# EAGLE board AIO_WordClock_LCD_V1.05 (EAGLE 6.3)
PROJECT_AUTHOR: C. Wille; PROJECT_COPYRIGHT: (c) 11/2012; PROJECT_REVISION: V1.05
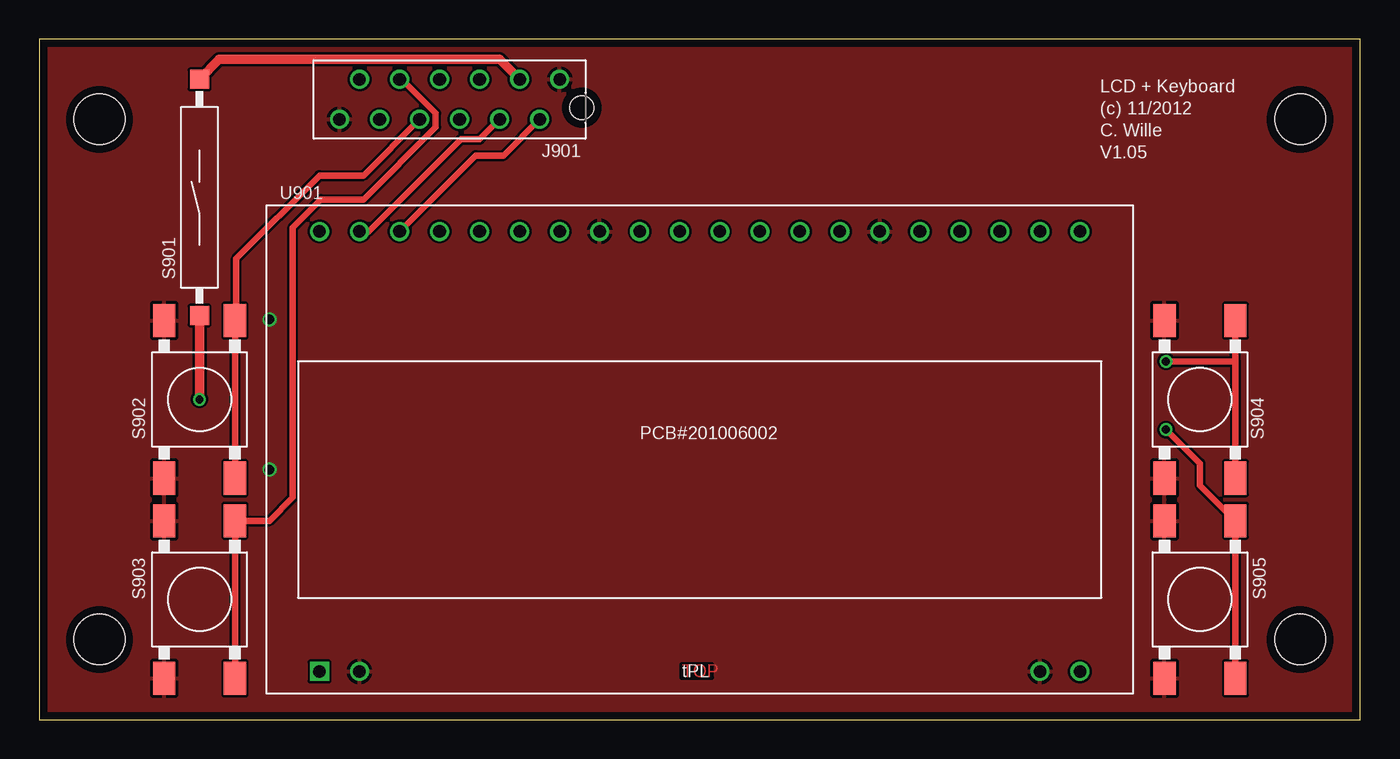
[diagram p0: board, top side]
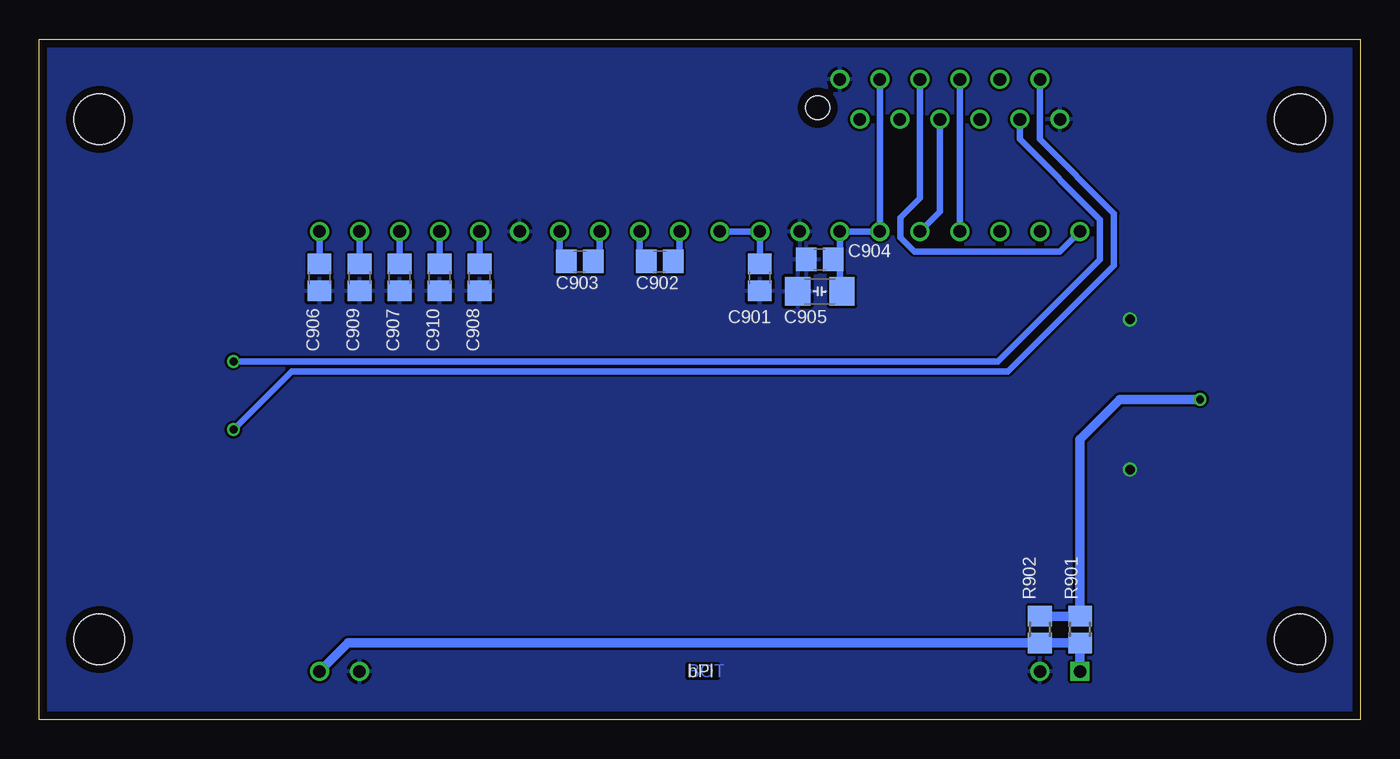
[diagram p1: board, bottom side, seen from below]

Size 83.82 x 43.18 mm. Coordinates in mm from the lower left corner, seen from the top.
Outline: 0,0 83.82,0 83.82,43.18 0,43.18 0,0
Copper layers (1*16): Top 0.035mm / dielectric 1.5mm / Bottom 0.035mm
Design rules "leiton": minimum track width 6mil, minimum drill 12mil, track to track 6mil, track to pad 6mil, pad to pad 6mil, via to via 6mil, smd to smd 6mil, copper to edge 20mil, drill to drill 8mil, minimum pad ring 8mil, minimum via ring 6mil, stop-mask expansion 3mil, vias tented up to drill 0mil, thermal gap 8mil
Holes 3.2 mm at 3.81,38.1 3.81,5.08 80.01,38.1 80.01,5.08

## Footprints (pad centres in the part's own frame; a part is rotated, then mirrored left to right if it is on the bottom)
C0805 = smd 1.3 x 1.5: 1 -0.85,0; 2 0.85,0
C1206 = smd 1.6 x 1.8: 1 -1.4,0; 2 1.4,0
MICRO-MATCH-12 = drill 0.8: 1 -6.985,-1.27; 2 -5.715,1.27; 3 -4.445,-1.27; 4 -3.175,1.27; 5 -1.905,-1.27; 6 -0.635,1.27; 7 0.635,-1.27; 8 1.905,1.27; 9 3.175,-1.27; 10 4.445,1.27; 11 5.715,-1.27; 12 6.985,1.27 | hole 1.5: -8.385,0.53
R0805@1 = smd 1.3 x 1.5: 1 -0.85,0; 2 0.85,0
MK16-X-2 = smd 1.2 x 1.2: 1 -7.5,0; 2 7.5,0
LSH1301 = smd 2.1 x 1.4: 1 -5,2.25; 2 5,2.25; 3 -5,-2.25; 4 5,-2.25
EA_DOGM132-5 = drill 0.8 square: 1 -24.13,-12.19 | drill 0.8: 2 -21.59,-12.19; 19 21.59,-12.19; 20 24.13,-12.19; 21 24.13,15.75; 22 21.59,15.75; 23 19.05,15.75; 24 16.51,15.75; 25 13.97,15.75; 26 11.43,15.75; 27 8.89,15.75; 28 6.35,15.75; 29 3.81,15.75; 30 1.27,15.75; 31 -1.27,15.75; 32 -3.81,15.75; 33 -6.35,15.75; 34 -8.89,15.75; 35 -11.43,15.75; 36 -13.97,15.75; 37 -16.51,15.75; 38 -19.05,15.75; 39 -21.59,15.75; 40 -24.13,15.75

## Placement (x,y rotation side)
C901  1E-6-1U-0805  [C0805]  38.1,28.07 270 bottom
C902  1E-6-1U-0805  [C0805]  44.45,29.08 180 bottom
C903  1E-6-1U-0805  [C0805]  49.53,29.08 180 bottom
C904  1E-6-1U-0805  [C0805]  34.29,29.21 180 bottom
C905  1E-6-10U-1206  [C1206]  34.29,27.18 180 bottom
C906  1E-6-1U-0805  [C0805]  66.04,28.07 270 bottom
C907  1E-6-1U-0805  [C0805]  60.96,28.07 270 bottom
C908  1E-6-1U-0805  [C0805]  55.88,28.07 270 bottom
C909  1E-6-1U-0805  [C0805]  63.5,28.07 270 bottom
C910  1E-6-1U-0805  [C0805]  58.42,28.07 270 bottom
J901  MICRO-MATCH-12  [MICRO-MATCH-12]  26.04,39.37 180 top
R901  1E0-3,3R-0805  [R0805@1]  17.78,5.71 270 bottom
R902  1E0-3,3R-0805  [R0805@1]  20.32,5.71 270 bottom
S901  MK16-SERIES  [MK16-X-2]  10.16,33.15 90 top
S902  LSH1301-9,5  [LSH1301]  10.16,20.32 90 top
S903  LSH1301-9,5  [LSH1301]  10.16,7.62 90 top
S904  LSH1301-9,5  [LSH1301]  73.66,20.32 90 top
S905  LSH1301-9,5  [LSH1301]  73.66,7.62 90 top
U901  EA_DOGM132B-5  [EA_DOGM132-5]  41.91,15.24 0 top

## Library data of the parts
C901-C904 C906-C910 = o.Capacitor 0603 0805 1206; MATERIAL: X7R; ORDER-MULTIPLE: 10; PACKAGE: 0805; SUPPLIER: Farnell; SUPPLIER-NUMBER: 145-8903; TOLERANCE: 10%; VAL: 1µ; VENDOR: Phycomp; VENDOR-NUMBER: 222291015663; VOLTAGE: 25V
C905 = o.Capacitor 0603 0805 1206; MATERIAL: X7R; ORDER-MULTIPLE: 1; PACKAGE: 1206; SUPPLIER: Reichelt; SUPPLIER-NUMBER: X5R-G1206 10/25; TOLERANCE: 10%; VAL: 10µ; VOLTAGE: 25V
J901 = o.Connectors.v5; SUPPLIER: Reichelt; SUPPLIER-NUMBER: MM FL 12G; VAL: Micro-MaTch 12; VENDOR: Tyco; VENDOR-NUMBER: 1-215079-2
R901 R902 = o.Resistor 0603 0805 1206; ORDER-MULTIPLE: 50; PACKAGE: 0805; SUPPLIER: Farnell; SUPPLIER-NUMBER: 933-3096; TOLERANCE: 1%; VAL: 3R3; VENDOR: multicomp; VENDOR-NUMBER: MC 0.1W 0805 3R3; WATTAGE: 0,1W
S901 = o.Switches; SUPPLIER: Farnell; SUPPLIER-NUMBER: 1079488; VAL: MK16-C-2; VENDOR: MEDER electronic; VENDOR-NUMBER: MK16-C-2
S902-S905 = o.Switches; SUPPLIER: Reichelt; SUPPLIER-NUMBER: TASTER9319; VAL: LSH 9.5 mm; VENDOR: Schurter; VENDOR-NUMBER: 1301.9319
U901 = o.Optical.v5; SUPPLIER: Reichelt; SUPPLIER-NUMBER: EA DOGM132B-5; VAL: EA DOGM132B-5; VENDOR: Electronic Assembly; VENDOR-NUMBER: EA DOGM132B-5

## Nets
A0: J901.2 U901.38
A+: R901.2 R902.2 U901.1 U901.20
BL: J901.9 S903.3 S903.4
BR: J901.11 S905.3 S905.4
CLK: J901.7 U901.37
CS#: J901.5 U901.40
DIN: J901.6 U901.36
GND: C901.2 C904.2 C905.2 C906.2 C907.2 C908.2 C909.2 C910.2 J901.1 J901.12 S902.1 S902.2 S903.1 S903.2 S904.1 S904.2 S905.1 S905.2 U901.2 U901.19 U901.26 U901.33
N$49: C903.2 U901.27
N$50: C903.1 U901.28
N$51: C902.2 U901.29
N$52: C902.1 U901.30
N$53: C901.1 U901.31 U901.32
RESET#: J901.4 U901.39
TL: J901.8 S902.3 S902.4
TR: J901.10 S904.3 S904.4
V0: C906.1 U901.21
V1: C909.1 U901.22
V2: C907.1 U901.23
V3: C910.1 U901.24
V4: C908.1 U901.25
VCC: C904.1 C905.1 J901.3 S901.2 U901.34 U901.35
VCC+: R901.1 R902.1 S901.1

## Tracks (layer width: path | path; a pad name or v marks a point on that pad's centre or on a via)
A0
  Top 0.406: U901.38 27.68,35.81 29.46,35.81 J901.2
A+
  Bottom 0.61: U901.1 R901.2 R902.2 64.22,4.87 U901.20
BL
  Top 0.406: S903.3 S903.4 14.6,12.62 16.08,14.1 16.08,31.24 17.86,33.02 20.57,33.02 25.15,37.59 25.15,38.48 22.99,40.64 J901.9
BR  (via drill 0.5)
  Top 0.406: v71.5,18.41 73.66,16.26 73.66,14.87 S905.4 S905.3
  Bottom 0.406: J901.11 20.32,36.83 15.62,32.13 15.62,28.83 22.35,22.1 67.82,22.1 v71.5,18.41
CLK
  Bottom 0.406: U901.37 J901.7
CS#
  Bottom 0.406: U901.40 19.05,29.72 28.27,29.72 29.16,30.61 29.16,31.88 27.94,33.1 J901.5
DIN
  Bottom 0.406: J901.6 26.67,32.26 U901.36
GND  (via drill 0.6)
  other vias: 14.61,25.4 14.61,15.88
  pour Bottom: 0,43.18 0,0 83.82,0 83.82,43.18
  pour Top: 0,43.18 0,0 83.82,0 83.82,43.18
N$49
  Bottom 0.406: U901.27 50.8,29.5 C903.2
N$50
  Bottom 0.406: U901.28 48.26,29.5 C903.1
N$51
  Bottom 0.406: U901.29 45.72,29.5 C902.2
N$52
  Bottom 0.406: U901.30 43.18,29.5 C902.1
N$53
  Bottom 0.406: C901.1 U901.32 U901.31
RESET#
  Top 0.406: U901.39 20.91,30.99 26.75,36.83 27.94,36.83 J901.4
TL
  Top 0.406: S902.3 S902.4 12.49,25.4 12.49,29.25 17.78,34.54 20.57,34.54 J901.8
TR  (via drill 0.5)
  Top 0.406: 75.91,22.73 S904.3 | 75.91,22.73 S904.4 | v71.5,22.73 75.91,22.73
  Bottom 0.406: J901.10 21.59,36.83 16.51,31.75 16.51,29.21 22.99,22.73 v71.5,22.73
V0
  Bottom 0.406: C906.1 U901.21
V1
  Bottom 0.406: C909.1 U901.22
V2
  Bottom 0.406: C907.1 U901.23
V3
  Bottom 0.406: C910.1 U901.24
V4
  Bottom 0.406: C908.1 U901.25
VCC
  Top 0.61: J901.3 29.21,41.91 11.42,41.91 S901.2
  Bottom 0.406: C905.1 33.02,27.18 33.02,29.21 | 33.02,29.21 U901.34 U901.35 J901.3 | 33.02,29.21 C904.1
VCC+  (via drill 0.5)
  Top 0.61: v10.16,20.32 S901.1
  Bottom 0.61: v10.16,20.32 15.24,20.32 17.78,17.78 R901.1 R902.1

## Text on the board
Top: TOP
Bottom: BOT
tPlace: LCD + Keyboard | PCB#201006002 | tPL
bPlace: bPl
